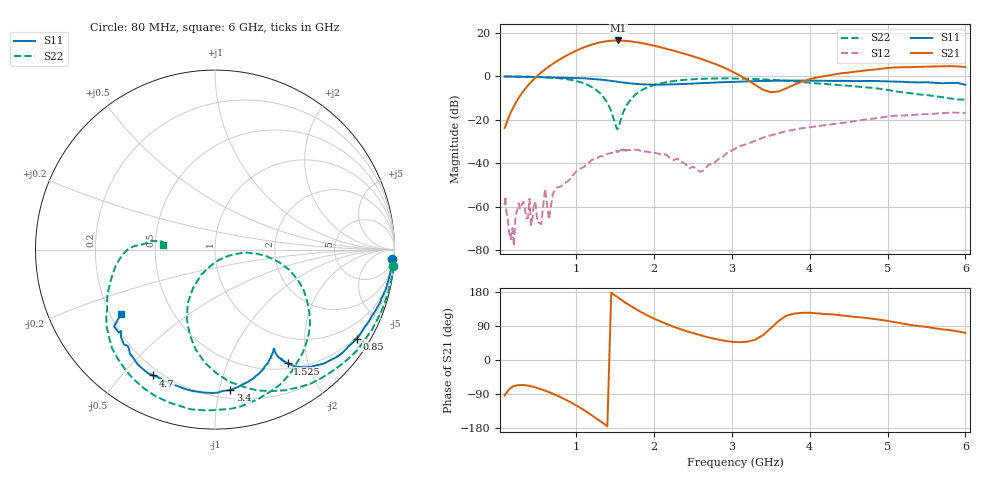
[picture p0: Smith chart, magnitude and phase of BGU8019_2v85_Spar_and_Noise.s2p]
! BGU8019,  Vcc= 2.85 V, Icc= 4.6025 mA
# MHz S MA R 50
!  Freq-MHz  S11-mag  S11-arg  S21-mag  S21-arg  S12-mag  S12-arg  S22-mag  S22-arg
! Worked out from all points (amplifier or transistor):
!   130 points, 80 MHz to 6 GHz, reference 50 ohm
!   highest |S21| = 16.5 dB at 1.54 GHz (marker M1)
!   |S21| within 3 dB of that: 1.112 GHz to 2.069 GHz (957.3 MHz wide, 60.2 % of centre)
!   unconditionally stable (mu >= 1): 125 MHz to 248.2 MHz; 265.8 MHz to 310.9 MHz; 326.5 MHz to end of sweep
!   at 480 MHz: K = 2.85, MAG = 21.9 dB, |S12| = -59.1 dB
!   at 1.615 GHz: K = 1.69, MAG = 20.2 dB, |S12| = -33.8 dB
!   at 6 GHz: K = 1.42, MAG = 6.7 dB, |S12| = -16.9 dB
!   lowest NFmin = 0.37 dB at 1.1 GHz
!   S11 on the Smith chart (normalised r, x): 80 MHz: 8, -35; 850 MHz: 0.45, -3.42; 1.525 GHz: 0.57, -1.68; 3.4 GHz: 0.26, -1.08; 4.7 GHz: 0.17, -0.61; 6 GHz: 0.24, -0.29
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80  0.988 -3.1  0.06477 -93.8  0.001097 168.2  0.9979 -5.2
200  0.9849 -8.0  0.2068 -68.8  0.000123 -31.5  0.9955 -13.5
260  0.9801 -10.4  0.3175 -66.2  0.001199 -35.0  0.9913 -17.5
550  0.9553 -21.3  1.227 -77.2  0.000394 -155.3  0.9634 -38.3
600  0.949 -22.9  1.443 -80.7  0.002581 -158.6  0.9522 -42.1
650  0.9462 -24.8  1.69 -84.8  0.0005071 -151.8  0.9411 -46.1
700  0.9405 -26.6  1.95 -88.9  0.001994 -122.3  0.93 -50.2
850  0.9321 -32.1  2.845 -103.2  0.00342 -157.3  0.8757 -63.5
1100  0.9014 -42.0  4.667 -132.2  0.008245 -175.0  0.6893 -89.3
1200  0.8777 -46.4  5.388 -145.8  0.01196 174.8  0.5673 -100.9
1350  0.8302 -52.2  6.282 -167.3  0.01457 153.8  0.3339 -117.0
1525  0.7522 -57.5  6.69 166.6  0.01933 130.6  0.06132 -68.1
1540  0.7474 -57.6  6.709 164.3  0.01919 129.0  0.06398 -45.7
1800  0.6608 -59.5  6.017 130.2  0.02046 93.9  0.4306 -15.3
2100  0.6434 -59.5  4.596 100.1  0.01573 57.2  0.7016 -41.8
2500  0.6823 -63.4  2.894 70.8  0.008372 -5.5  0.8562 -71.1
3100  0.7592 -75.9  1.052 46.9  0.02471 -141.3  0.8893 -106.7
3400  0.787 -83.8  0.4905 65.5  0.03868 -162.0  0.8527 -122.3
4100  0.7935 -102.3  0.9488 122.9  0.07119 161.2  0.6862 -151.2
4700  0.7811 -116.2  1.359 111.6  0.1007 142.1  0.5638 -170.2
5100  0.759 -126.3  1.605 99.6  0.1238 127.4  0.454 177.7
6000  0.6373 -145.5  1.637 71.6  0.1437 100.4  0.2917 174.7
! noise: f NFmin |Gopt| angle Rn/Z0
1000  0.4065  0.6392  29.93  0.1946
1250  0.4081  0.6276  31.99  0.1896
1505  0.4528  0.5904  42.05  0.1941
1535  0.4669  0.6102  41.86  0.1924
1560  0.4687  0.6124  42.37  0.1871
1590  0.4805  0.6301  42.3  0.1844
1620  0.5071  0.6025  44.33  0.1856
1645  0.4884  0.602  45.02  0.1829
1900  0.538  0.6103  47.01  0.2063
2200  0.6581  0.5367  59.15  0.181
